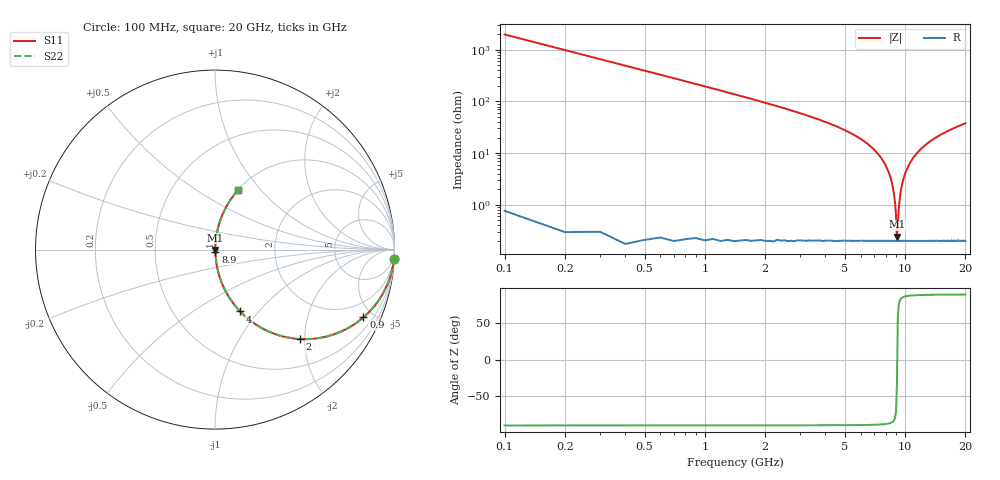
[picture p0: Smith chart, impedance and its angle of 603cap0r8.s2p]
! AVX Thin Film Operation		Date: November 2004
! Description: Accu-P® Series, Thin Film, SMD, RF Capacitor
! Part Number: 06035J0R8ABT
! 50 MHz  -  10.05 GHz
! Serial Measurements
# hz S db R 50
!	S11		S21		S12		S22
!	dB	Phase	dB	Phase	dB	Phase	dB	Phase
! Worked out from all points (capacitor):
!   200 points, 100 MHz to 20 GHz, reference 50 ohm
!   read as one part in series: C = 800 fF near 200 MHz
!   lowest |Z| = 241 mohm at 9.1 GHz (marker M1)
!   series resonance near 9.128 GHz, so ESL is about 380 pH
!   S11 on the Smith chart (normalised r, x): 100 MHz: 1, -40; 900 MHz: 1.00, -4.38; 2 GHz: 1.00, -1.89; 4 GHz: 1.00, -0.80; 8.9 GHz: 1.00, -0.02; 20 GHz: 1.00, +0.76
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1e8  -0.01 -2.9  -25.98 87.1  -25.98 87.1  -0.01 -2.9
2e8  -0.04 -5.7  -19.99 84.2  -19.99 84.2  -0.04 -5.7
4e8  -0.17 -11.4  -14.09 78.6  -14.09 78.6  -0.17 -11.4
9e8  -0.83 -24.5  -7.63 65.4  -7.63 65.4  -0.83 -24.5
2e9  -3.26 -46.5  -2.79 43.4  -2.79 43.4  -3.26 -46.5
3.5e9  -7.22 -63.9  -0.93 25.8  -0.93 25.8  -7.22 -63.9
4e9  -8.58 -67.9  -0.67 21.9  -0.67 21.9  -8.58 -67.9
6.8e9  -17.80 -81.7  -0.09 7.4  -0.09 7.4  -17.80 -81.7
8.2e9  -26.61 -84.9  -0.03 2.7  -0.03 2.7  -26.61 -84.9
8.6e9  -31.70 -84.1  -0.02 1.5  -0.02 1.5  -31.70 -84.1
8.9e9  -39.02 -79.1  -0.02 0.6  -0.02 0.6  -39.02 -79.1
9e9  -43.79 -71.7  -0.02 0.4  -0.02 0.4  -43.79 -71.7
9.1e9  -52.37 -33.9  -0.02 0.1  -0.02 0.1  -52.37 -33.9
9.2e9  -48.06 59.5  -0.02 -0.2  -0.02 -0.2  -48.06 59.5
9.3e9  -41.56 75.7  -0.02 -0.5  -0.02 -0.5  -41.56 75.7
9.5e9  -35.15 82.5  -0.02 -1.0  -0.02 -1.0  -35.15 82.5
9.8e9  -30.18 84.5  -0.02 -1.8  -0.02 -1.8  -30.18 84.5
1.01e10  -27.11 84.9  -0.03 -2.5  -0.03 -2.5  -27.11 84.9
1.13e10  -20.61 83.4  -0.06 -5.3  -0.06 -5.3  -20.61 83.4
1.34e10  -15.46 79.6  -0.14 -9.7  -0.14 -9.7  -15.46 79.6
1.67e10  -11.41 74.0  -0.34 -15.6  -0.34 -15.6  -11.41 74.0
2e10  -9.04 69.0  -0.60 -20.7  -0.60 -20.7  -9.04 69.0
